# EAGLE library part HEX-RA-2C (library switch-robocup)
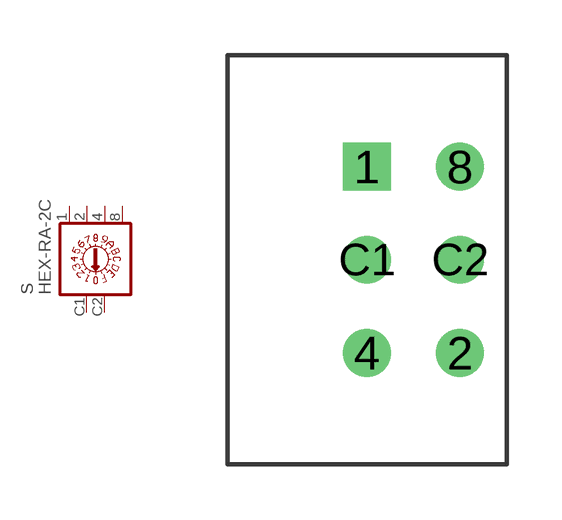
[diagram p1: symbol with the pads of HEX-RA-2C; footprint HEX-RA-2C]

Designator prefix S

## HEX-RA-2C  [HEX-RA-2C]
1  1  pas
2  2  pas
4  4  pas
8  8  pas
C1  C1  pas
C2  C2  pas

## Footprint HEX-RA-2C (pad centres in mm)
drill 0.8 square: 1 0,2.54
drill 0.8: 2 2.54,-2.54; 4 0,-2.54; 8 2.54,2.54; C1 0,0; C2 2.54,0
